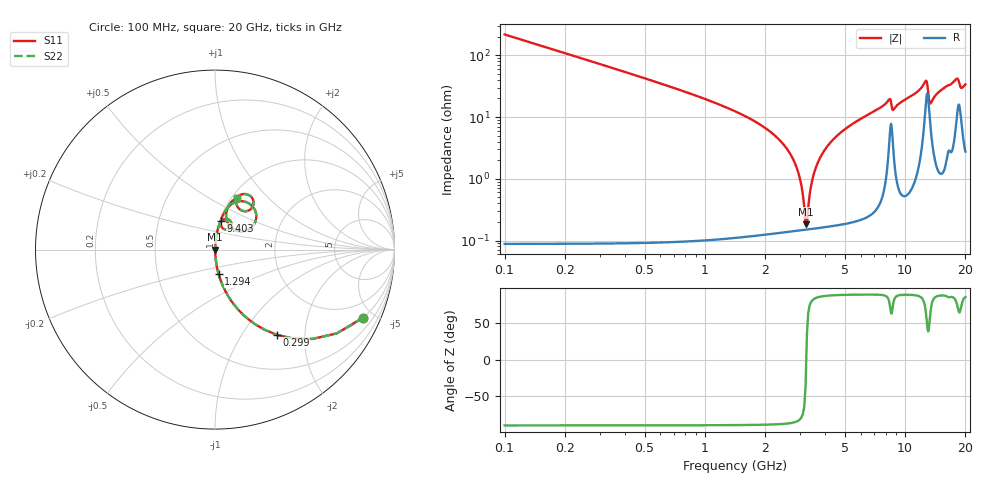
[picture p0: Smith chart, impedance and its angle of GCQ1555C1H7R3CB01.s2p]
!Murata Part Number: GCQ1555C1H7R3CB01
!These Parameters are Measured in Series Mode Connection
!Data Generated on Mar 13, 2026
!  o--ll--o
!Port1  Port2
!  o------o
!Operation Temp=25[degC], DC Bias Voltage=0[V]
!Freq. Start=100[MHz] Stop=20[GHz] 401[Steps]
# Hz S RI R 50
!Freq.(Hz) S11(Real) S11(Imag) S21(Real) S21(Imag) S12(Real) S12(Imag) S22(Real) S22(Imag)
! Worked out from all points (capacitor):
!   401 points, 100 MHz to 20 GHz, reference 50 ohm
!   read as one part in series: C = 7.3 pF near 199.5 MHz
!   lowest |Z| = 183 mohm at 3.184 GHz (marker M1)
!   series resonance near 3.209 GHz, so ESL is about 340 pH
!   S11 on the Smith chart (normalised r, x): 100 MHz: 1.00, -4.36; 299 MHz: 1.00, -1.45; 1.294 GHz: 1.00, -0.28; 9.403 GHz: 1.01, +0.34; 20 GHz: 1.06, +0.67
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1e8  0.8258 -0.3791  0.1742 0.3791  0.1742 0.3791  0.8258 -0.3791
2.99e8  0.3434 -0.4742  0.6566 0.4742  0.6566 0.4742  0.3434 -0.4742
5.975e8  0.111 -0.3128  0.889 0.3128  0.889 0.3128  0.111 -0.3128
1.294e9  0.0205 -0.138  0.9795 0.138  0.9795 0.138  0.0205 -0.138
2.63725e9  0.0021 -0.0268  0.9979 0.0268  0.9979 0.0268  0.0021 -0.0268
2.93575e9  0.00159 -0.0121  0.9984 0.0121  0.9984 0.0121  0.00159 -0.0121
3.1845e9  0.0015 -0.00105  0.9985 0.00105  0.9985 0.00105  0.0015 -0.00105
3.284e9  0.00152 0.00313  0.9985 -0.00313  0.9985 -0.00313  0.00152 0.00313
3.43325e9  0.00163 0.00919  0.9984 -0.00919  0.9984 -0.00919  0.00163 0.00919
3.7815e9  0.00211 0.0225  0.9979 -0.0225  0.9979 -0.0225  0.00211 0.0225
4.3785e9  0.00359 0.0431  0.9964 -0.0431  0.9964 -0.0431  0.00359 0.0431
6.7665e9  0.0159 0.1145  0.9841 -0.1145  0.9841 -0.1145  0.0159 0.1145
8.30875e9  0.0634 0.1711  0.9366 -0.1711  0.9366 -0.1711  0.0634 0.1711
8.70675e9  0.0465 0.1162  0.9535 -0.1162  0.9535 -0.1162  0.0465 0.1162
9.40325e9  0.0332 0.162  0.9668 -0.162  0.9668 -0.162  0.0332 0.162
1.005e10  0.0409 0.1848  0.9591 -0.1848  0.9591 -0.1848  0.0409 0.1848
1.2637e10  0.1999 0.2498  0.8001 -0.2498  0.8001 -0.2498  0.1999 0.2498
1.338325e10  0.0844 0.1285  0.9156 -0.1285  0.9156 -0.1285  0.0844 0.1285
1.67165e10  0.1183 0.2833  0.8817 -0.2833  0.8817 -0.2833  0.1183 0.2833
1.8408e10  0.2149 0.2586  0.7851 -0.2586  0.7851 -0.2586  0.2149 0.2586
1.9005e10  0.1444 0.22  0.8556 -0.22  0.8556 -0.22  0.1444 0.22
2e10  0.1213 0.288  0.8787 -0.288  0.8787 -0.288  0.1213 0.288
